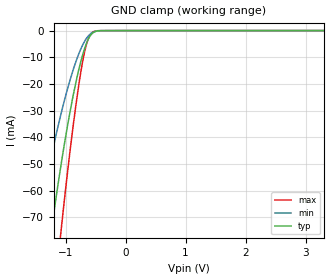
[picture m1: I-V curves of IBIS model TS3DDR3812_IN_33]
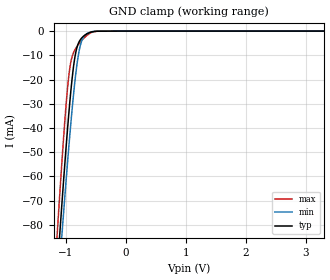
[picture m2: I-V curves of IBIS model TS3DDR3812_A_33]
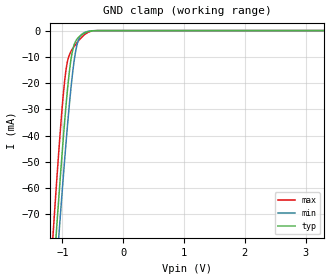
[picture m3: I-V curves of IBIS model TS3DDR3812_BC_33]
| TEXAS INSTRUMENTS INCORPORATED
| Standard Linear and Logic Group / High Volume Linear
| IBIS Model of TS3DDR3812
| 12 CHANNEL, 1:2 MUX/DEMUX SWITCH FOR DDR3 APPLICATIONS
| This file contains package information for the following:
|  QFN 42-pin (RUA) package as [Component] TS3DDR3812_RUA
| This device can be powered at the following Vccs:
|  3.3 volt Vcc
| This file provides unique models under the [Model Selector] for each Vcc.
| For operation at a specific Vcc, select the appropriate model after each
| [Model Selector] keyword.
[IBIS Ver]   3.2
[Comment char]  |_char
[File Name]   ts3ddr3812.ibs
[File Rev]   1.1 | x_die
[Date]   September 2, 2010
[Source]   Data created from TI-SPICE simulations at TI-SLL/HVL.
   The following is an IBIS list for the TS3DDR3812.
   Please contact sllibis@ti.com with questions and
   comments concerning SLL IBIS models.
[Notes]   Revision_History:
   1.1 - swapped pins 39&40 (B1&C1) and 41&42 (B0&C0)
[Disclaimer]
| This model is designed as an aid for customers of Texas Instruments.
| TI and its licensors and suppliers make no warranties, either expressed
| or implied, with respect to this  model, including the warranties of
| merchantability or fitness for a particular purpose. The model is
| provided solely on an "as is" basis. The entire risk as to its quality
| and performance is with the customer.
[Copyright]
| (C) Copyright 2010 Texas Instruments Incorporated. All rights reserved.
| Component TS3DDR3812_RUA 42-PIN QFN
[Component]   TS3DDR3812_RUA
[Manufacturer]   Texas Instruments, Inc.
[Package]
|   typ   min   max
R_pkg   1.024e-01   6.263e-02   1.372e-01
L_pkg   2.245e-09   1.300e-09   3.156e-09
C_pkg   2.642e-13   1.816e-13   3.573e-13
[Pin]   signal_name   model_name   R_pin   L_pin   C_pin
1   VCC   POWER   1.358e-01   3.026e-09   2.905e-13
2   A0   TS3DDR3812_A_33   1.290e-01   2.862e-09   3.263e-13
3   A1   TS3DDR3812_A_33   1.158e-01   2.549e-09   3.115e-13
4   A2   TS3DDR3812_A_33   1.029e-01   2.247e-09   2.774e-13
5   A3   TS3DDR3812_A_33   9.101e-02   1.968e-09   2.469e-13
6   A4   TS3DDR3812_A_33   8.034e-02   1.720e-09   2.222e-13
7   A5   TS3DDR3812_A_33   7.122e-02   1.509e-09   1.996e-13
8   EN   TS3DDR3812_IN_33   6.616e-02   1.393e-09   1.889e-13
9   SEL1   TS3DDR3812_IN_33   6.303e-02   1.321e-09   1.857e-13
10   SEL2   TS3DDR3812_IN_33   6.449e-02   1.355e-09   1.889e-13
11   A6   TS3DDR3812_A_33   7.023e-02   1.486e-09   2.008e-13
12   A7   TS3DDR3812_A_33   7.899e-02   1.688e-09   2.192e-13
13   A8   TS3DDR3812_A_33   8.950e-02   1.933e-09   2.417e-13
14   A9   TS3DDR3812_A_33   1.007e-01   2.195e-09   2.662e-13
15   A10   TS3DDR3812_A_33   1.120e-01   2.460e-09   2.982e-13
16   A11   TS3DDR3812_A_33   1.254e-01   2.775e-09   3.215e-13
17   VCC   POWER   1.345e-01   2.996e-09   2.925e-13
18   C11   TS3DDR3812_BC_33   1.365e-01   3.140e-09   3.562e-13
19   B11   TS3DDR3812_BC_33   1.292e-01   2.864e-09   2.970e-13
20   C10   TS3DDR3812_BC_33   1.292e-01   2.862e-09   2.969e-13
21   B10   TS3DDR3812_BC_33   1.366e-01   3.137e-09   3.562e-13
22   C9   TS3DDR3812_BC_33   1.348e-01   2.997e-09   3.023e-13
23   B9   TS3DDR3812_BC_33   1.211e-01   2.668e-09   3.116e-13
24   C8   TS3DDR3812_BC_33   1.100e-01   2.405e-09   2.864e-13
25   B8   TS3DDR3812_BC_33   9.879e-02   2.142e-09   2.577e-13
26   C7   TS3DDR3812_BC_33   8.940e-02   1.921e-09   2.377e-13
27   B7   TS3DDR3812_BC_33   7.884e-02   1.675e-09   2.186e-13
28   C6   TS3DDR3812_BC_33   6.993e-02   1.468e-09   2.000e-13
29   B6   TS3DDR3812_BC_33   6.414e-02   1.334e-09   1.876e-13
30   VCC   POWER   6.263e-02   1.300e-09   1.816e-13
31   C5   TS3DDR3812_BC_33   6.461e-02   1.345e-09   1.858e-13
32   B5   TS3DDR3812_BC_33   7.083e-02   1.489e-09   2.017e-13
33   C4   TS3DDR3812_BC_33   7.997e-02   1.701e-09   2.210e-13
34   B4   TS3DDR3812_BC_33   9.067e-02   1.951e-09   2.406e-13
35   C3   TS3DDR3812_BC_33   1.002e-01   2.174e-09   2.611e-13
36   B3   TS3DDR3812_BC_33   1.115e-01   2.440e-09   2.898e-13
37   C2   TS3DDR3812_BC_33   1.225e-01   2.700e-09   3.136e-13
38   B2   TS3DDR3812_BC_33   1.356e-01   3.015e-09   3.026e-13
39   B1   TS3DDR3812_BC_33   1.372e-01   3.154e-09   3.573e-13
40   C1   TS3DDR3812_BC_33   1.299e-01   2.879e-09   2.983e-13
41   B0   TS3DDR3812_BC_33   1.299e-01   2.881e-09   2.983e-13
42   C0   TS3DDR3812_BC_33   1.372e-01   3.156e-09   3.567e-13
[Series Switch Groups]
| Function Group States
On  1 /   | A0-A5->B0-B5 SEL1 LOW, EN HIGH
   | B0-B5->A0-A5 SEL1 LOW, EN HIGH
On  2 /   | A0-A5->C0-C5 SEL1 HIGH, EN HIGH
   | C0-C5->A0-A5 SEL1 HIGH, EN HIGH
On  3 /   | A6-A11->B6-B11 SEL2 LOW, EN HIGH
   | B6-B11->A6-A11 SEL2 LOW, EN HIGH
On  4 /   | A6-A11->C6-C11 SEL2 HIGH, EN HIGH
   | C6-C11->A6-A11 SEL2 HIGH, EN HIGH
Off 1 2 3 4  /   | EN LOW
[Series Pin Mapping]   pin_2   model_name   function_table_group
2   42   TS3DDR3812_A_33_S   1
3   40   TS3DDR3812_A_33_S   1
4   38   TS3DDR3812_A_33_S   1
5   36   TS3DDR3812_A_33_S   1
6   34   TS3DDR3812_A_33_S   1
7   32   TS3DDR3812_A_33_S   1
42   2   TS3DDR3812_BC_33_S   1
40   3   TS3DDR3812_BC_33_S   1
38   4   TS3DDR3812_BC_33_S   1
36   5   TS3DDR3812_BC_33_S   1
34   6   TS3DDR3812_BC_33_S   1
32   7   TS3DDR3812_BC_33_S   1
2   41   TS3DDR3812_A_33_S   2
3   39   TS3DDR3812_A_33_S   2
4   37   TS3DDR3812_A_33_S   2
5   35   TS3DDR3812_A_33_S   2
6   33   TS3DDR3812_A_33_S   2
7   31   TS3DDR3812_A_33_S   2
41   2   TS3DDR3812_BC_33_S   2
39   3   TS3DDR3812_BC_33_S   2
37   4   TS3DDR3812_BC_33_S   2
35   5   TS3DDR3812_BC_33_S   2
33   6   TS3DDR3812_BC_33_S   2
31   7   TS3DDR3812_BC_33_S   2
11   29   TS3DDR3812_A_33_S   3
12   27   TS3DDR3812_A_33_S   3
13   25   TS3DDR3812_A_33_S   3
14   23   TS3DDR3812_A_33_S   3
15   21   TS3DDR3812_A_33_S   3
16   19   TS3DDR3812_A_33_S   3
29   11   TS3DDR3812_BC_33_S   3
27   12   TS3DDR3812_BC_33_S   3
25   13   TS3DDR3812_BC_33_S   3
23   14   TS3DDR3812_BC_33_S   3
21   15   TS3DDR3812_BC_33_S   3
19   16   TS3DDR3812_BC_33_S   3
11   28   TS3DDR3812_A_33_S   4
12   26   TS3DDR3812_A_33_S   4
13   24   TS3DDR3812_A_33_S   4
14   22   TS3DDR3812_A_33_S   4
15   20   TS3DDR3812_A_33_S   4
16   18   TS3DDR3812_A_33_S   4
28   11   TS3DDR3812_BC_33_S   4
26   12   TS3DDR3812_BC_33_S   4
24   13   TS3DDR3812_BC_33_S   4
22   14   TS3DDR3812_BC_33_S   4
20   15   TS3DDR3812_BC_33_S   4
18   16   TS3DDR3812_BC_33_S   4
[Model]   TS3DDR3812_A_33_S
Model_type  Series_switch
| variable   typ   min   max
C_comp   0   0   0
[Temperature Range]   40   100   -40
| Ambient temperature   25   85   -40
[Voltage range]   3.3   3   3.6
[On]
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[Off]
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[Model]   TS3DDR3812_BC_33_S
Model_type  Series_switch
| variable   typ   min   max
C_comp   0   0   0
[Temperature Range]   40   100   -40
| Ambient temperature   25   85   -40
[Voltage range]   3.3   3   3.6
[On]
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[Off]
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| Models and submodels in the file (5): TS3DDR3812_IN_33 (Input), TS3DDR3812_A_33_S (Series_switch), TS3DDR3812_A_33 (Terminator), TS3DDR3812_BC_33_S (Series_switch), TS3DDR3812_BC_33 (Terminator)
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| Model TS3DDR3812_IN
| Model TS3DDR3812_A
| Model TS3DDR3812_A_S
| Model TS3DDR3812_BC
| Model TS3DDR3812_BC_S
[Model]   TS3DDR3812_IN_33
Model_type  Input
Vinl=0.8
Vinh=2.0
| variable   typ   min   max
C_comp   3.00pF   2.63pF   3.38pF
[Temperature Range]   40   100   -40
| Ambient temperature   25   85   -40
[Voltage range]   3.3   3   3.6
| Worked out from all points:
|   GND clamp passes 1 mA (typ) near -0.55 V on its own axis
[GND Clamp]
| TS3DDR3812_IN_33
|   Voltage   I(typ)   I(min)   I(max)
-3.3V     -514.7mA   -370.1mA   -672.6mA
-1.49V    -118.9mA   -76.58mA   -172.7mA
-1.45V    -111.6mA   -71.63mA   -162.7mA
-1.24V    -75.5mA    -47.55mA   -111.9mA
-1.08V    -51.01mA   -31.63mA   -76.14mA
-1.065V   -48.88mA   -30.26mA   -72.96mA
-885mV    -25.72mA   -15.57mA   -37.8mA
-745mV    -11.56mA   -6.876mA   -15.45mA
-695mV    -7.603mA   -4.542mA   -9.294mA
-640mV    -4.141mA   -2.557mA   -4.326mA
-530mV    -630.9uA   -478.8uA   -382.7uA
3.3V      208.2pA    780.8pA    25.79pA
[Model]   TS3DDR3812_A_33
Model_type  Terminator
| variable   typ   min   max
C_comp   1.59pF   1.51pF   1.70pF
| C_tri-state   1.59pF   1.51pF   1.70pF
[Temperature Range]   40   100   -40
| Ambient temperature   25   85   -40
[Voltage range]   3.3   3   3.6
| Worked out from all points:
|   GND clamp passes 1 mA (typ) near -0.64 V on its own axis
[GND Clamp]
| TS3DDR3812_A_33
|   Voltage   I(typ)   I(min)   I(max)
-3.3V     -974.3mA   -942.8mA   -1.003A
-1.15V    -101.5mA   -112.9mA   -86.27mA
-1.135V   -96.07mA   -107.7mA   -80.41mA
-1.105V   -85.29mA   -97.55mA   -68.86mA
-1.09V    -79.98mA   -92.5mA    -63.2mA
-1.065V   -71.23mA   -84.17mA   -53.96mA
-955mV    -35.52mA   -49.34mA   -19.6mA
-915mV    -24.45mA   -37.75mA   -12.61mA
-860mV    -12.57mA   -23.46mA   -8.314mA
-765mV    -3.842mA   -6.639mA   -4.75mA
-645mV    -1.086mA   -1.02mA    -1.723mA
3.3V      742.1pA    25.37nA    110.5pA
[Model]   TS3DDR3812_BC_33
Model_type  Terminator
| variable   typ   min   max
C_comp   1.29pF   1.22pF   1.40pF
| C_tri-state   1.29pF   1.22pF   1.40pF
[Temperature Range]   40   100   -40
| Ambient temperature   25   85   -40
[Voltage range]   3.3   3   3.6
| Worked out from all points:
|   GND clamp passes 1 mA (typ) near -0.64 V on its own axis
[GND Clamp]
| TS3DDR3812_BC_33
|   Voltage   I(typ)   I(min)   I(max)
-3.3V     -891.9mA   -884.3mA   -896.3mA
-1.15V    -93.43mA   -107.6mA   -76.19mA
-1.1V     -76.78mA   -91.33mA   -59.13mA
-1.06V    -63.81mA   -78.59mA   -46.05mA
-1.045V   -59.05mA   -73.88mA   -41.34mA
-950mV    -30.94mA   -45.39mA   -16.52mA
-910mV    -20.87mA   -34.38mA   -11.04mA
-855mV    -10.36mA   -20.87mA   -7.779mA
-800mV    -4.956mA   -10.39mA   -5.811mA
-755mV    -3.104mA   -5.006mA   -4.441mA
-625mV    -822uA     -617uA     -1.349mA
3.3V      658.5pA    25.27nA    62.15pA
